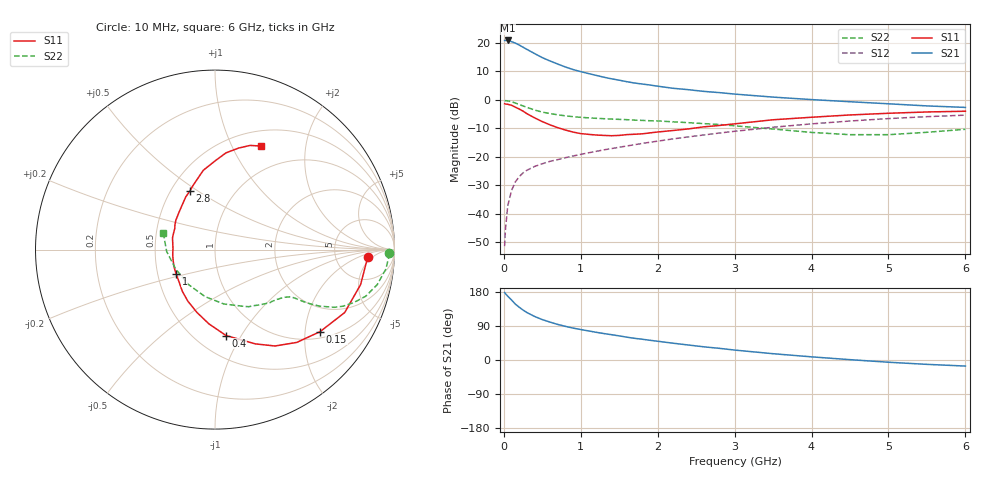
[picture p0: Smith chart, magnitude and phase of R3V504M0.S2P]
! SIEMENS Small Signal Semiconductors
! BFR181
! Si NPN RF Bipolar Junction Transistor in SOT23
! VCE = 0.5 V  IC = 4 mA
! Common Emitter S-Parameters:  May  1996
# GHz  S  MA  R  50
!  f  S11  S21  S12  S22
! GHz  MAG  ANG  MAG  ANG  MAG  ANG  MAG  ANG
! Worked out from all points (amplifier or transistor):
!   36 points, 10 MHz to 6 GHz, reference 50 ohm
!   highest |S21| = 20.8 dB at 50 MHz (marker M1)
!   |S21| within 3 dB of that: start of sweep to 291.1 MHz
!   unconditionally stable (mu >= 1): 783.6 MHz to 4.928 GHz; 5.579 GHz to end of sweep
!   at 250 MHz: K = 0.44, MSG = 22.1 dB, |S12| = -25.6 dB
!   at 1.4 GHz: K = 1.21, MAG = 9.5 dB, |S12| = -17.1 dB
!   at 6 GHz: K = 1.01, MAG = 0.8 dB, |S12| = -5.4 dB
!   S11 on the Smith chart (normalised r, x): 10 MHz: 12, -3; 150 MHz: 1.18, -2.40; 400 MHz: 0.69, -0.86; 1 GHz: 0.62, -0.18; 2.8 GHz: 0.62, +0.46; 6 GHz: 0.68, +1.30
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0.01  0.8534 -2.7  11.02 178.0  0.0027 89.0  0.9707 -1.2
0.02  0.8453 -5.2  11 175.4  0.0051 85.1  0.9683 -2.6
0.05  0.8344 -13.5  11.02 168.6  0.0136 82.2  0.9587 -6.4
0.1  0.8032 -25.9  10.51 158.4  0.0257 76.1  0.9247 -12.2
0.15  0.7427 -38.0  9.883 147.4  0.0363 69.0  0.8789 -17.2
0.2  0.6893 -48.6  9.159 139.2  0.0449 65.1  0.8275 -20.9
0.25  0.6326 -58.1  8.381 131.8  0.0522 61.3  0.7809 -23.8
0.3  0.5709 -66.9  7.68 125.2  0.0582 59.5  0.7386 -25.8
0.4  0.4826 -82.7  6.481 114.9  0.0677 55.5  0.6623 -28.4
0.5  0.4146 -94.8  5.502 106.6  0.0755 54.0  0.6085 -29.7
0.6  0.364 -106.1  4.81 100.0  0.0833 53.6  0.5743 -30.4
0.7  0.3247 -117.8  4.249 93.9  0.0892 53.3  0.546 -30.9
0.8  0.2949 -128.2  3.772 88.8  0.0964 53.4  0.5238 -31.2
1  0.2553 -148.3  3.125 80.4  0.1102 54.5  0.4928 -32.3
1.1  0.2479 -156.8  2.893 76.8  0.1174 55.0  0.4831 -33.2
1.6  0.2454 164.8  2.079 60.2  0.1551 55.7  0.4482 -38.0
2.2  0.2896 133.6  1.594 44.3  0.2063 54.2  0.4109 -47.2
2.8  0.3545 113.4  1.339 30.8  0.2612 50.7  0.3694 -59.5
3.5  0.4467 98.4  1.116 16.6  0.3304 44.4  0.3071 -80.7
4.5  0.5426 83.5  0.926 0.9  0.4248 32.8  0.2445 -127.1
5.5  0.6124 71.4  0.782 -11.5  0.5063 19.7  0.2693 -177.7
6  0.6307 66.2  0.736 -16.0  0.5389 12.8  0.304 161.8
